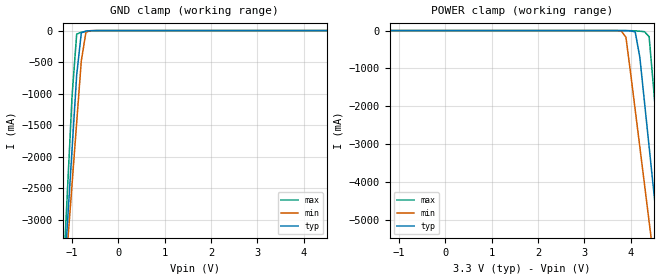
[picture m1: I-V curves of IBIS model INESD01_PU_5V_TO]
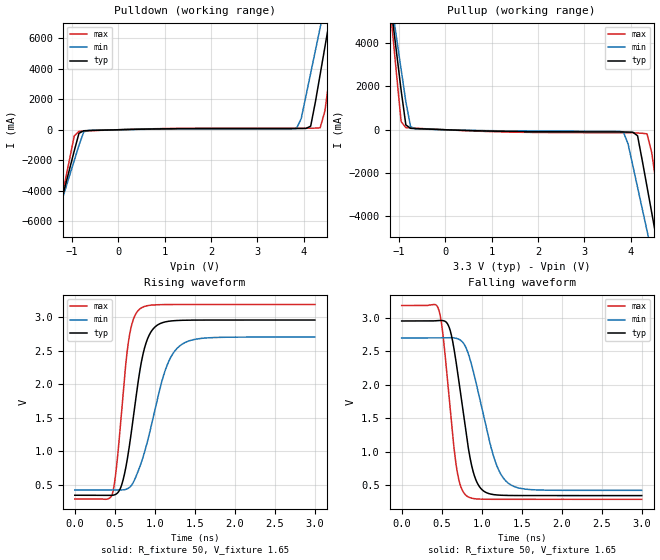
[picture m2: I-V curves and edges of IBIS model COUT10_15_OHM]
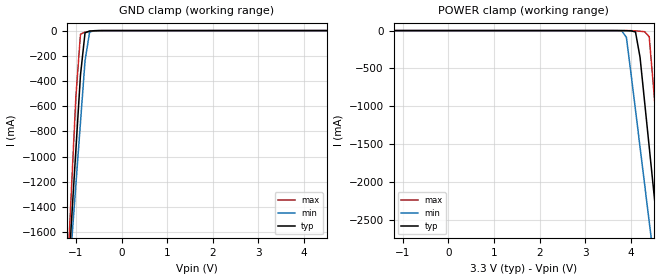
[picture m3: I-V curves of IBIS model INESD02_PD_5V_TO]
|   This file is an IBIS representation of the   |
|   Integrated Devices Technology, Inc.   |
|   ICS83115   |
|   LOW SKEW, 1-TO-16 LVCMOS/LVTTL FANOUT BUFFER   |
[IBIS Ver]   4.1
[File name]   83115_3v3.ibs
[File Rev]   1.0
[Date]   6 Apr 2009 | Last modified
|   Feb 28 2006 | Generated
[Source]   Originated at Integrated Devices Technology, Inc.
[Disclaimer]
IDT hereby grants the user of this IBIS model a non-exclusive,
nontransferable license to use this IBIS model under the following terms.
Before using this IBIS model, the user should read this license.
If the user does not accept these terms,  the IBIS model should be
returned to IDT within 30 days.
   The user is granted this license only to use the IBIS model and
is not granted rights to sell, load, rent, lease or license the IBIS
model in whole or in part, or in modified form to anyone other than
user. User may modify the IBIS model to suit its specific
applications but rights to derivative works and such modifications
shall belong to IDT.
   This IBIS model is provided on an "AS IS" basis and IDT makes
absolutely no warranty with respect to the information contained
herein. IDT DISCLAIMS AND CUSTOMER WAIVES ALL WARRANTIES, EXPRESS
OR IMPLIED, INCLUDING WARRANTIES OF MERCHANTABILITY OR FITNESS FOR
A PARTICULAR PURPOSE. The entire risk as to quality and performance
is with the Customer. ACCORDINGLY, IN NO EVENT SHALL THE COMPANY BE
LIABLE FOR ANY DAMAGES, WHETHER IN CONTRACT OR TORT,INCLUDING ANY
LOST PROFITS OR OTHER INCIDENTAL, CONSEQUENTIAL, EXEMPLARY, OR
PUNITIVE DAMAGES ARISING OUT OF THE USE OR APPLICATION OF THE IBIS
model provided in this package. Further, IDT reserves the right to
make changes without notice to any product herein to improve
reliability, function, or design. IDT does not convey any license
under patent rights or any other intellectual property rights,
including those of third parties.
   IDT is not obligated to provide maintenance or support
for the licensed IBIS model.
[Copyright]   Copyright 2006 by Integrated Device Technology, Inc.
[Component]   ICS83115BR
[Manufacturer] Integrated Devices Technology, Inc.
[Package]
|SSOP 20 Lead
|   typ   min   max
R_pkg   66.7m   54.1m   79.3m
L_pkg   2.262nH   1.601nH   2.922nH
C_pkg   0.329pF   0.232pF   0.427pF
[Pin] signal_name   model_name   R_pin   L_pin   C_pin
1   OE1   INESD01_PU_5V_TO   79.3m   2.922n   0.427p
2   Q0   COUT10_15_OHM   75.1m   2.702n   0.395p
3   Q1   COUT10_15_OHM   70.9m   2.482n   0.362p
4   Q2   COUT10_15_OHM   66.7m   2.262n   0.329p
5   VDD   POWER   62.5m   2.041n   0.297p
6   VDD   POWER   58.3m   1.821n   0.264p
7   Q3   COUT10_15_OHM   54.1m   1.601n   0.232p
8   Q4   COUT10_15_OHM   54.1m   1.601n   0.232p
9   GND   GND   58.3m   1.821n   0.264p
10   GND   GND   62.5m   2.041n   0.297p
11   Q5   COUT10_15_OHM   66.7m   2.262n   0.329p
12   Q6   COUT10_15_OHM   70.9m   2.482n   0.362p
13   Q7   COUT10_15_OHM   75.1m   2.702n   0.395p
14   IN   INESD02_PD_5V_TO   79.3m   2.922n   0.427p
15   OE0   INESD01_PU_5V_TO   79.3m   2.922n   0.427p
16   Q8   COUT10_15_OHM   75.1m   2.702n   0.395p
17   Q9   COUT10_15_OHM   70.9m   2.482n   0.362p
18   Q10   COUT10_15_OHM   66.7m   2.262n   0.329p
19   GND   GND   62.5m   2.041n   0.297p
20   GND   GND   58.3m   1.821n   0.264p
21   Q11   COUT10_15_OHM   54.1m   1.601n   0.232p
22   Q12   COUT10_15_OHM   54.1m   1.601n   0.232p
23   VDD   POWER   58.3m   1.821n   0.264p
24   VDD   POWER   62.5m   2.041n   0.297p
25   Q13   COUT10_15_OHM   66.7m   2.262n   0.329p
26   Q14   COUT10_15_OHM   70.9m   2.482n   0.362p
27   Q15   COUT10_15_OHM   75.1m   2.702n   0.395p
28   OE2   INESD01_PU_5V_TO   79.3m   2.922n   0.427p
| Models and submodels in the file (3): INESD01_PU_5V_TO (Input), COUT10_15_OHM (Output), INESD02_PD_5V_TO (Input)
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[Model]   INESD01_PU_5V_TO
Model_type   Input
Polarity   Non-Inverting
Vinl = 1.4V
Vinh = 1.85V
|   typ   min   max
C_comp   2pF   1.5pF   2.5pF
|   typ   min   max
[Voltage range]  3.3V   3.135V   3.465V
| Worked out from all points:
|   GND clamp passes 1 mA (typ) near -0.53 V on its own axis
[GND_clamp]
|Voltage   I(typ)   I(min)   I(max)
-3.3V     -29.05A    -25.05A    -35.74A
-1.2V     -4.246A    -4.402A    -4.061A
-1.1V     -3.066A    -3.421A    -2.553A
-1V       -1.886A    -2.44A     -1.044A
-900mV    -707.2mA   -1.46A     -57.45mA
-800mV    -35.64mA   -480.8mA   -24.42mA
-700mV    -7.042mA   -24.07mA   -13.3mA
-600mV    -2.123mA   -1.734mA   -4.923mA
6.6V      64.3uA     84.42uA    57.85uA
[POWER_clamp]
|Voltage   I(typ)   I(min)   I(max)
-3.3V     64.3uA     80.4uA     60.89uA
3.8V      -415.9uA   -8.87mA    -79.9uA
3.9V      -2.123mA   -177.6mA   -256.3uA
4.1V      -35.64mA   -2.097A    -7.435mA
4.2V      -707.2mA   -3.077A    -16.94mA
4.3V      -1.886A    -4.058A    -29.28mA
4.4V      -3.066A    -5.04A     -160.2mA
4.5V      -4.246A    -6.022A    -1.572A
4.6V      -5.426A    -7.005A    -3.08A
4.7V      -6.607A    -7.988A    -4.589A
4.8V      -7.788A    -8.971A    -6.098A
6.6V      -29.05A    -26.68A    -33.25A
[Model]   COUT10_15_OHM
Model_type   Output
Polarity   Non-Inverting
Vmeas = 1.65
Rref = 50
Cref = 0
Vref = 1.65
|   typ   min   max
C_comp   2pF   1.5pF   2.5pF
|   typ   min   max
[Voltage range]  3.3V   3.135V   3.465V
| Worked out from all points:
|   slope of the pulldown table from 0 to 0.495 V, typ, clamps not added: 13.8 ohm
|   slope of the pullup table from 0 to 0.495 V, typ, clamps not added: 13.7 ohm
|   rising waveform, R_fixture 50, V_fixture 1.65: 20-80 % time 196ps typ, 298ps min, 137ps max; typ from 0.341 V to 2.96 V
|   falling waveform, R_fixture 50, V_fixture 1.65: 20-80 % time 193ps typ, 277ps min, 144ps max; typ from 2.96 V to 0.341 V
[pulldown]
|Voltage   I (typ)   I (min)   I (max)
-3.3V     -29.16A    -25.15A    -35.86A
-1.463V   -7.429A    -7.049A    -8.123A
-1.361V   -6.221A    -6.044A    -6.58A
-952.6mV  -1.39A     -2.025A    -405.5mA
-850.5mV  -234.5mA   -1.022A    -103.8mA
-646.4mV  -52.93mA   -43.23mA   -68.97mA
3.844V    79.54mA    85.8mA     101.9mA
4.151V    235.2mA    3.716A     103.7mA
4.355V    3.628A     6.703A     124.5mA
4.559V    7.219A     9.692A     3.517A
4.763V    10.81A     12.68A     8.113A
6.6V      43.31A     39.72A     49.65A
[pullup]
|Voltage   I (typ)   I (min)   I (max)
-3.3V     43.25A     37.27A     53.27A
-1.157V   5.426A     5.787A     4.935A
-952.6mV  1.827A     2.793A     380.1mA
-850.5mV  222.5mA    1.296A     95.37mA
-748.5mV  65.22mA    142.1mA    80.97mA
-646.4mV  53.41mA    42.85mA    69.61mA
3.844V    -102.2mA   -100.2mA   -139.3mA
4.151V    -277.4mA   -2.661A    -152.1mA
4.355V    -2.633A    -4.664A    -188.6mA
4.559V    -5.043A    -6.67A     -2.6A
4.763V    -7.453A    -8.676A    -5.681A
6.6V      -29.16A    -26.75A    -33.4A
[Ramp]
|   typ   min   max
dV/dt_r   2.093/0.305n   1.826/0.463n   2.325/0.212n
dV/dt_f   2.098/0.289n   1.829/0.416n   2.333/0.215n
[Rising Waveform]
R_fixture = 50
V_fixture = 1.65
V_fixture_max = 1.73
V_fixture_min = 1.57
C_fixture = 0.0p
| Time   typ   min   max
0s        340.7mV    419.1mV    284.7mV
465ps     339.1mV    419.2mV    348.2mV
514.6ps   356.7mV    418.6mV    695.2mV
576.6ps   464.6mV    417.6mV    1.477V
672.7ps   1.005V     448.4mV    2.651V
812.2ps   2.197V     766.3mV    3.121V
973.4ps   2.816V     1.47V      3.179V
1.144ns   2.931V     2.253V     3.186V
1.324ns   2.951V     2.581V     3.187V
2.998ns   2.955V     2.701V     3.187V
[Falling Waveform]
R_fixture = 50
V_fixture = 1.65
V_fixture_max = 1.73
V_fixture_min = 1.57
C_fixture = 0.0p
| Time   typ   min   max
0s        2.955V     2.701V     3.187V
461.9ps   2.963V     2.701V     3.127V
511.5ps   2.961V     2.701V     2.792V
589ps     2.873V     2.705V     1.86V
682ps     2.322V     2.696V     785mV
809.1ps   1.236V     2.539V     338.5mV
970.3ps   475.6mV    1.818V     288.3mV
1.163ns   353.1mV    873.6mV    285mV
1.327ns   342.9mV    531mV      284.7mV
2.998ns   340.7mV    419.1mV    284.7mV
[Model]   INESD02_PD_5V_TO
Model_type   Input
Polarity   Non-Inverting
Vinl = 0.8V
Vinh = 2.0V
|   typ   min   max
C_comp   2pF   1.5pF   2.5pF
|   typ   min   max
[Voltage range]  3.3V   3.135V   3.465V
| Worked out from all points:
|   GND clamp passes 1 mA (typ) near -0.60 V on its own axis
[GND_clamp]
|Voltage I(typ)   I(min)   I(max)
-3.3V     -14.52A    -12.53A    -17.87A
-1.2V     -2.123A    -2.201A    -2.031A
-1.1V     -1.533A    -1.71A     -1.276A
-1V       -943mA     -1.22A     -522mA
-900mV    -353.5mA   -729.8mA   -28.69mA
-800mV    -17.79mA   -240.3mA   -12.18mA
-700mV    -3.491mA   -12mA      -6.618mA
-600mV    -1.033mA   -835uA     -2.43mA
6.6V      128.6uA    160.8uA    121.8uA
[POWER_clamp]
|Voltage   I(typ)   I(min)   I(max)
-3.3V     128.6uA    156.8uA    124.8uA
3.8V      -180.1uA   -4.403mA   -11.05uA
3.9V      -1.033mA   -88.76mA   -99.86uA
4.1V      -17.79mA   -1.048A    -3.685mA
4.2V      -353.5mA   -1.539A    -8.437mA
4.3V      -943mA     -2.029A    -14.61mA
4.4V      -1.533A    -2.52A     -80.08mA
4.5V      -2.123A    -3.011A    -786mA
4.6V      -2.713A    -3.502A    -1.54A
4.7V      -3.303A    -3.994A    -2.295A
4.8V      -3.894A    -4.485A    -3.049A
6.6V      -14.52A    -13.34A    -16.62A
